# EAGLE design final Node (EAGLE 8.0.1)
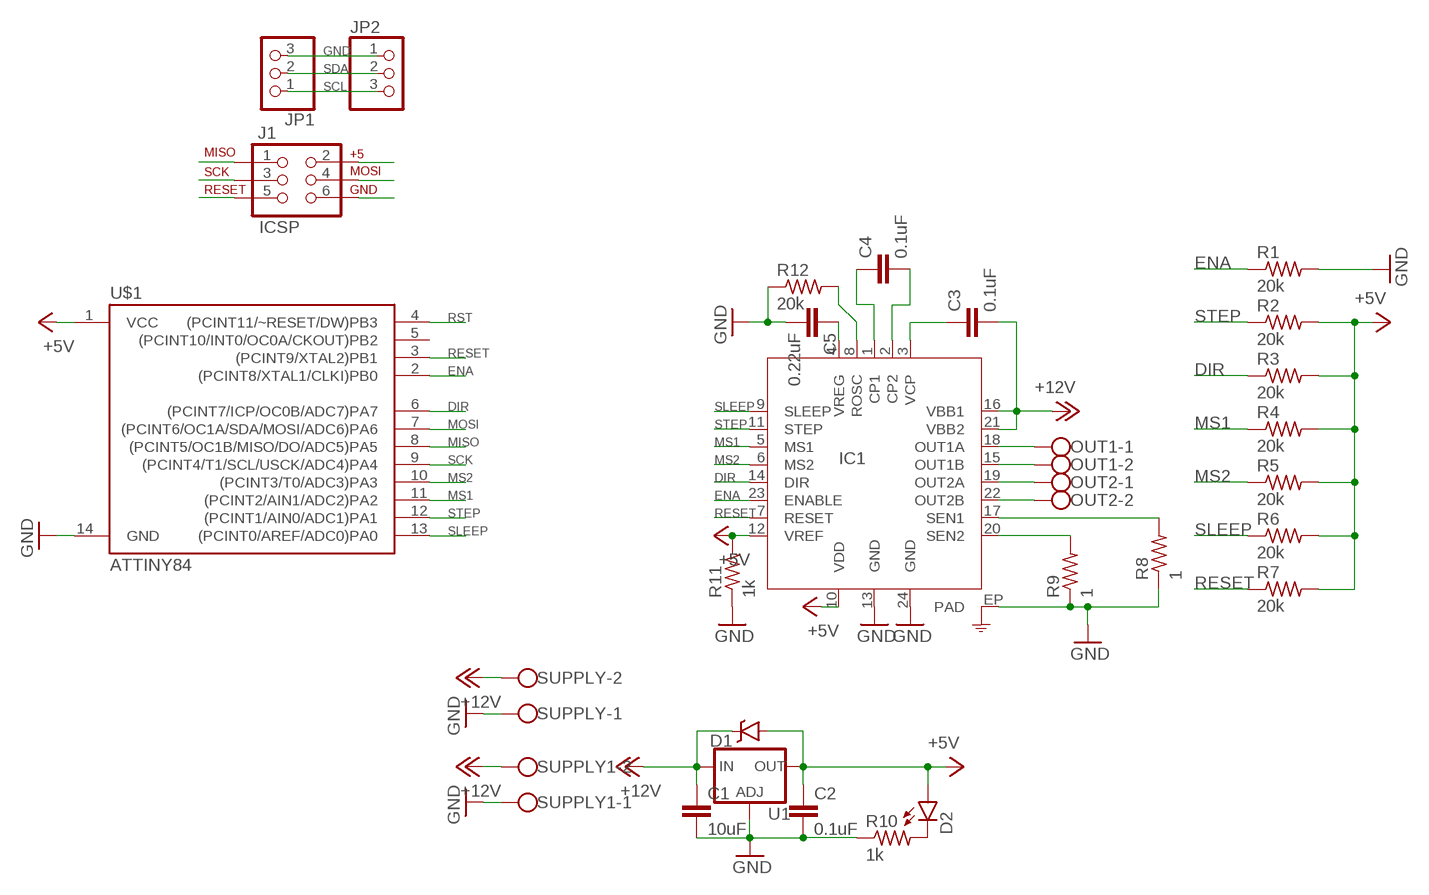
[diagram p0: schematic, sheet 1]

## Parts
C1  10uF  C-EUC1206  [C1206]
C2  0.1uF  C-EUC1206  [C1206]
C3  0.1uF  C-EUC1206  [C1206]
C4  0.1uF  C-EUC1206  [C1206]
C5  0.22uF  C-EUC1206  [C1206]
D1  DIODE-SCHOTTKY-BAT20J  [SOD-323]
D2  LED1206  [LED-1206]
IC1  A4982  [TSSOP-24]
J1  ICSP  AVR_SPI_PRG_6OFFSET_PADS  [2X3_OFFSET]
JP1  PINHD-1X3  [1X03]
JP2  PINHD-1X3  [1X03]
OUT1  W237-102  [W237-102]
OUT2  W237-102  [W237-102]
R1  20k  R-US_R1206  [R1206]
R2  20k  R-US_R1206  [R1206]
R3  20k  R-US_R1206  [R1206]
R4  20k  R-US_R1206  [R1206]
R5  20k  R-US_R1206  [R1206]
R6  20k  R-US_R1206  [R1206]
R7  20k  R-US_R1206  [R1206]
R8  1  R-US_R1206  [R1206]
R9  1  R-US_R1206  [R1206]
R10  1k  R-US_R1206  [R1206]
R11  1k  R-US_R1206  [R1206]
R12  20k  R-US_R1206  [R1206]
SUPPLY  W237-102  [W237-102]
SUPPLY1  W237-102  [W237-102]
U1  V_REG_317SMD  [SOT223]
U$1  ATTINY84  [SO14]

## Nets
5V: J1.2
+5V: C2.1 D1.A D2.A IC1.10(VDD) IC1.12(VREF) R2.2 R3.2 R4.2 R5.2 R6.2 R7.2 R11.2 U1.2(OUT) U$1.1(VCC)
+12V: C1.1 C3.2 D1.C IC1.16(VBB1) IC1.21(VBB2) SUPPLY1.2 SUPPLY.2 U1.3(IN)
DIR: IC1.14(DIR) R3.1 U$1.6((PCINT7/ICP/OC0B/ADC7)PA7)
ENA: IC1.23(ENABLE) R1.1 U$1.2((PCINT8/XTAL1/CLKI)PB0)
GND: C1.2 C2.2 C5.2 IC1.13(GND) IC1.24(GND) IC1.EP(PAD) J1.6 JP1.3 JP2.1 R1.2 R8.1 R9.1 R10.1 R11.1 R12.1 SUPPLY1.1 SUPPLY.1 U1.1(ADJ) U$1.14(GND)
MISO: J1.1 U$1.8((PCINT5/OC1B/MISO/DO/ADC5)PA5)
MOSI: J1.4 JP1.2 JP2.2 U$1.7((PCINT6/OC1A/SDA/MOSI/ADC6)PA6)
MS1: IC1.5(MS1) R4.1 U$1.11((PCINT2/AIN1/ADC2)PA2)
MS2: IC1.6(MS2) R5.1 U$1.10((PCINT3/T0/ADC3)PA3)
N$1: C3.1 IC1.3(VCP)
N$2: D2.C R10.2
N$8: C4.2 IC1.2(CP2)
N$9: C4.1 IC1.1(CP1)
N$11: C5.1 IC1.4(VREG)
N$12: IC1.8(ROSC) R12.2
OU1B: IC1.15(OUT1B) OUT1.2
OUT1A: IC1.18(OUT1A) OUT1.1
OUT2A: IC1.19(OUT2A) OUT2.1
OUT2B: IC1.22(OUT2B) OUT2.2
RESET: IC1.7(RESET) R7.1 U$1.3((PCINT9/XTAL2)PB1)
RST: J1.5 U$1.4((PCINT11/~RESET/DW)PB3)
SCK: J1.3 JP1.1 JP2.3 U$1.9((PCINT4/T1/SCL/USCK/ADC4)PA4)
SEN1: IC1.17(SEN1) R8.2
SEN2: IC1.20(SEN2) R9.2
SLEEP: IC1.9(SLEEP) R6.1 U$1.13((PCINT0/AREF/ADC0)PA0)
STEP: IC1.11(STEP) R2.1 U$1.12((PCINT1/AIN0/ADC1)PA1)
Unconnected: U$1.5((PCINT10/INT0/OC0A/CKOUT)PB2)

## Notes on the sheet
- SDA
- SCL

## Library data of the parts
C1-C5 = resistor:C-EU: CAPACITOR, European symbol
D1 = SparkFun-DiscreteSemi:DIODE-SCHOTTKY: Schottky diodes in SFE's production catalog; PROD_ID: DIO-11623; VALUE: BAT20J
D2 = SparkFun-LED:LED: LEDs
IC1 = SparkFun-DigitalIC:A4982: IC Full Bridge Motor Driver DMOS Microstepping Driver with Translator And Overcurrent Protection VBB 35V 2A
J1 = SparkFun-Connectors:AVR_SPI_PRG_6: AVR ISP 6 Pin This is the reduced ISP connector for AVR programming. Common on Arduino. This footprint will take up less PCB space and can be used with a 10-pin to 6-pin adapter such as SKU: BOB-08508 **Special note about "TEST_POINT" package. The stop mask is on the top side, so if you want your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
JP1 JP2 = pinhead:PINHD-1X3: PIN HEADER
OUT1 OUT2 SUPPLY SUPPLY1 = con-wago-500:W237-102: WAGO SCREW CLAMP; MPN: 237-102; OC_FARNELL: unknown; OC_NEWARK: 70K9898
R1-R12 = resistor:R-US_: RESISTOR, American symbol
U1 = SparkFun-PowerIC:V_REG_317: Voltage Regulator Standard LM317 adjustable voltage regulator. AOI (Adjust Output Input). Google 'LM317 Calculator' for easy to use app to get the two resistor values needed. 240/720 for 5V output. 240/390 for 3.3V output. Spark Fun Electronics SKU : COM-00527
U$1 = SparkFun-DigitalIC:ATTINY84: Atmel 14-pin 2/4/8kB flash uC; PROD_ID: IC-11285

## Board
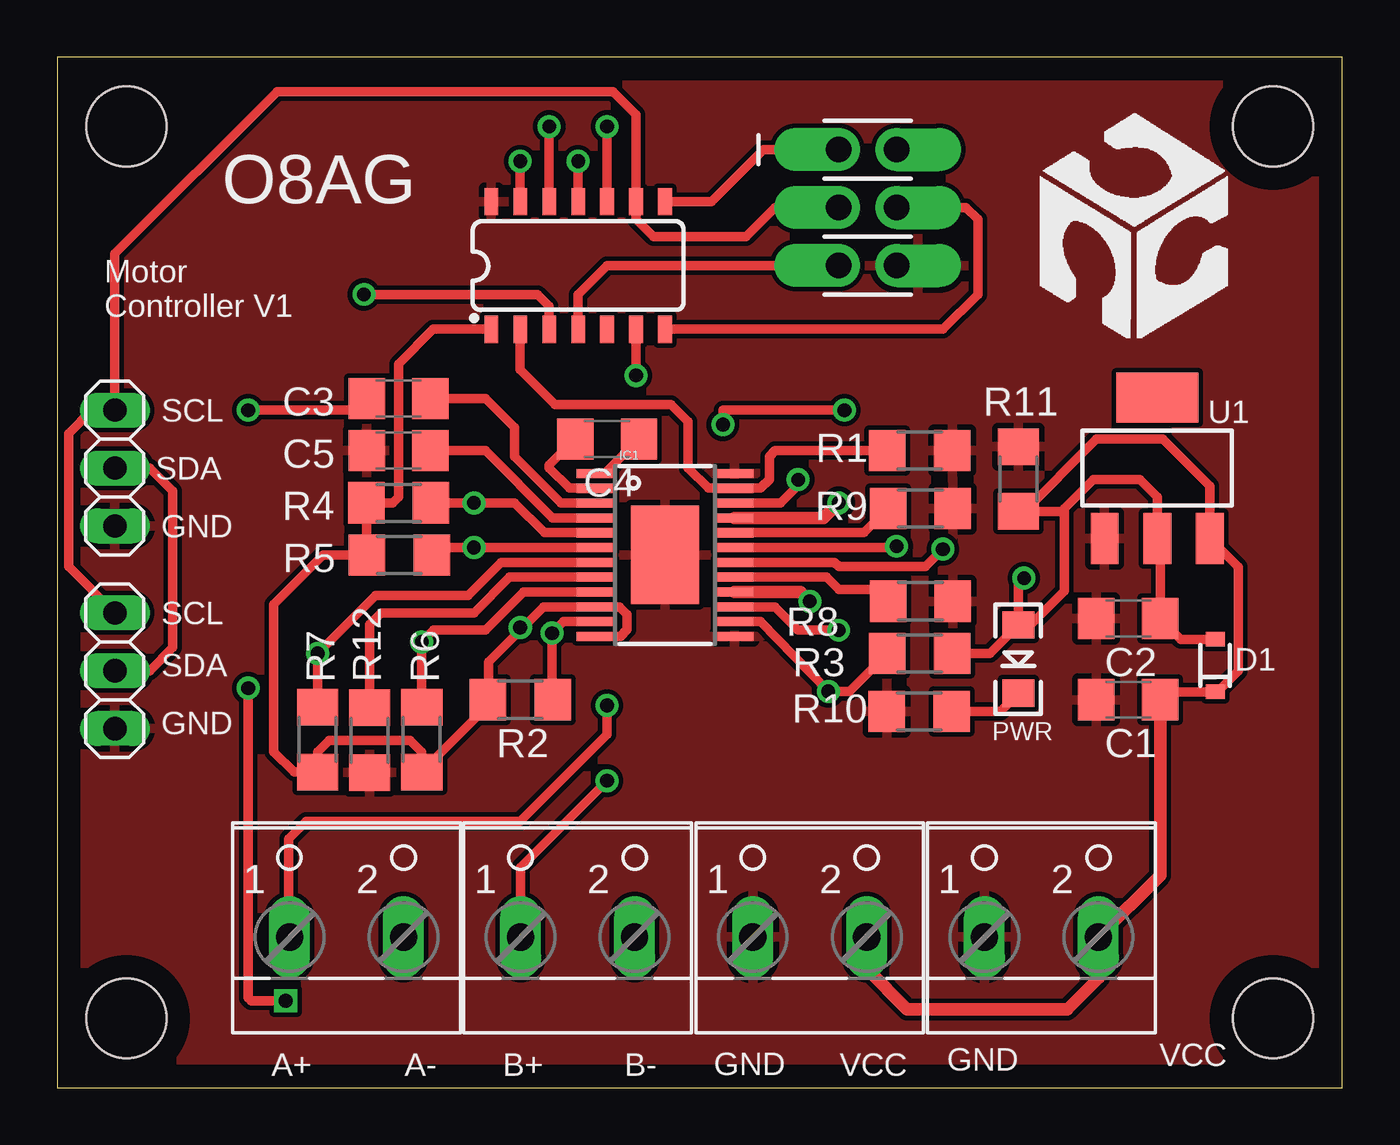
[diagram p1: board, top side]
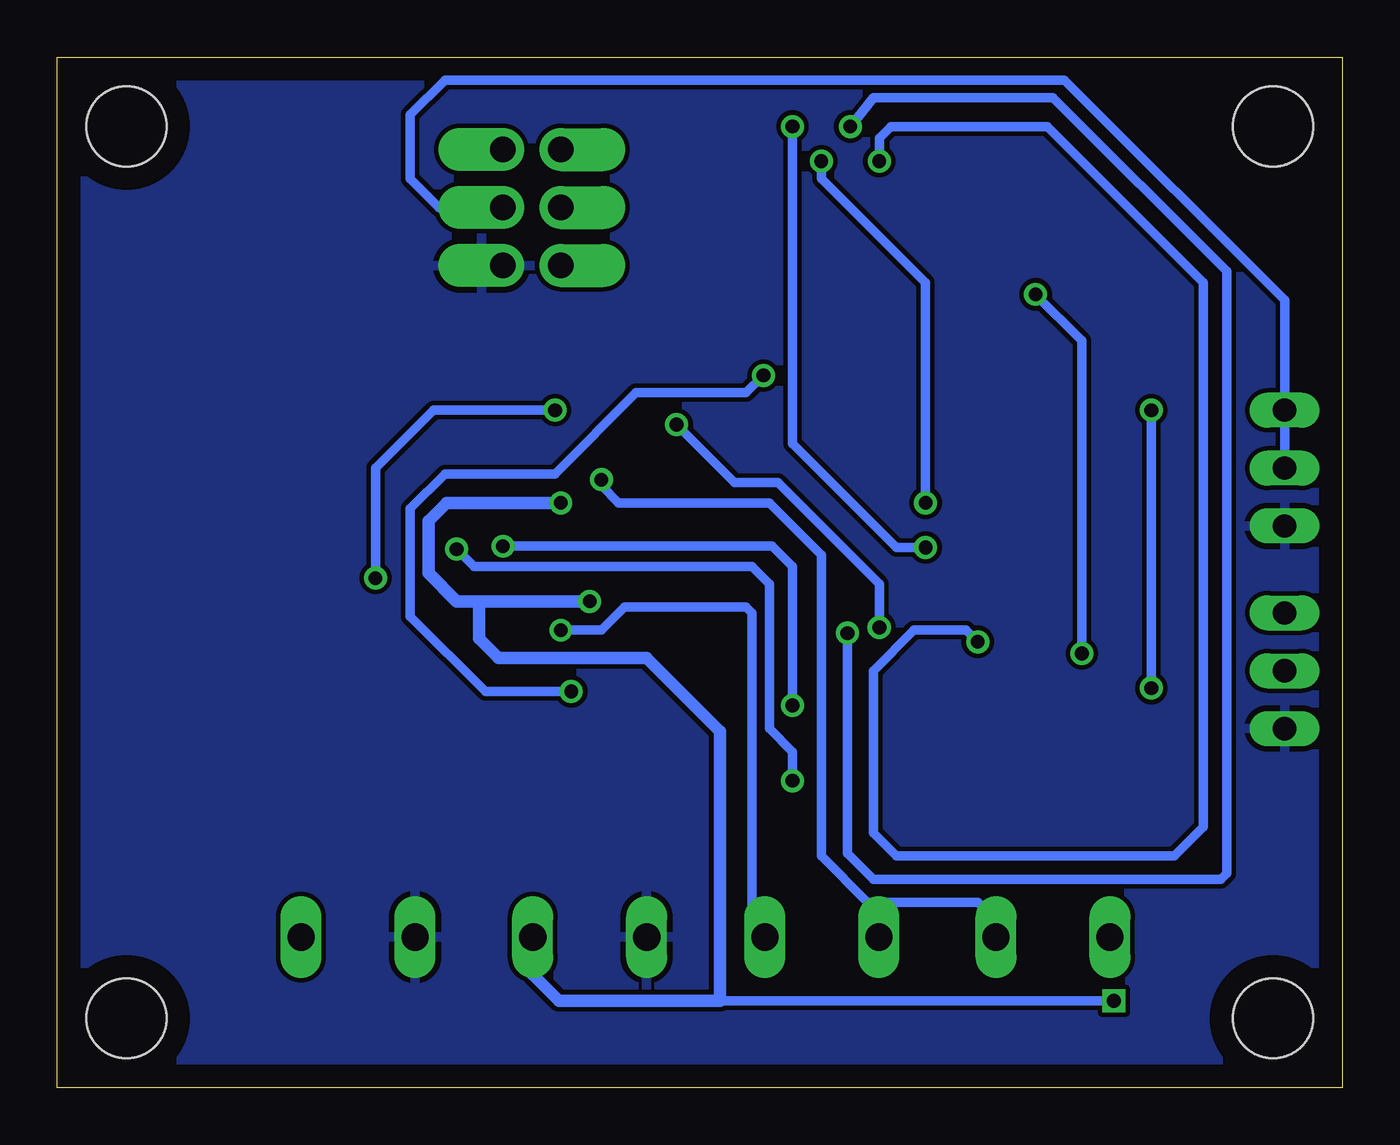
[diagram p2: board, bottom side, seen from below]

Size 56.39 x 45.21 mm. Coordinates in mm from the lower left corner, seen from the top.
Outline: 0,0 56.39,0 56.39,45.21 0,45.21 0,0
Copper layers (1*16): Top 0.035mm / dielectric 1.5mm / Bottom 0.035mm
Design rules "default *": minimum track width 16mil, minimum drill 24mil, track to track 8mil, track to pad 8mil, pad to pad 8mil, via to via 8mil, smd to smd 8mil, copper to edge 40mil, drill to drill 8mil, minimum pad ring 10mil, minimum via ring 8mil, stop-mask expansion 4mil, vias tented up to drill 0mil, thermal gap 10mil
Holes 3.5 mm at 3.05,3.05 53.34,3.05 53.34,42.16 3.05,42.16

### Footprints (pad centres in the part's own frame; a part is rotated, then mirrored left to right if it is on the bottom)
C1206 = smd 1.6 x 1.8: 1 -1.4,0; 2 1.4,0
SOD-323 = smd 0.63 x 0.83: A 1.15,0; C -1.15,0
LED-1206 = smd 1.2 x 1.4: A -1.5,0; C 1.5,0
TSSOP-24 = smd 0.4 x 1.65: 1 -3.575,-3.05; 2 -2.925,-3.05; 3 -2.275,-3.05; 4 -1.625,-3.05; 5 -0.975,-3.05; 6 -0.325,-3.05; 7 0.325,-3.05; 8 0.975,-3.05; 9 1.625,-3.05; 10 2.275,-3.05; 11 2.925,-3.05; 12 3.575,-3.05; 13 3.575,3.05; 14 2.925,3.05; 15 2.275,3.05; 16 1.625,3.05; 17 0.975,3.05; 18 0.325,3.05; 19 -0.325,3.05; 20 -0.975,3.05; 21 -1.625,3.05; 22 -2.275,3.05; 23 -2.925,3.05; 24 -3.575,3.05 | smd 4.32 x 3: EP 0,0
2X3_OFFSET = drill 1.118 pad 1.88 offset: 1 -2.54,-1.27; 2 -2.54,1.27; 3 0,-1.27; 4 0,1.27; 5 2.54,-1.27; 6 2.54,1.27
1X03 = drill 1.016 long: 1 -2.54,0; 2 0,0; 3 2.54,0
W237-102 = drill 1.194 long: 1 -2.5,-1.27; 2 2.5,-1.27
R1206 = smd 1.6 x 1.803: 1 -1.422,0; 2 1.422,0
SOT223 = smd 1.219 x 2.235: 1 -2.311,-3.099; 2 0,-3.099; 3 2.311,-3.099 | smd 3.6 x 2.2: 4 0,3.099
SO14 = smd 0.6 x 1.2: 1 -3.81,-2.8; 2 -2.54,-2.8; 3 -1.27,-2.8; 4 0,-2.8; 5 1.27,-2.8; 6 2.54,-2.8; 7 3.81,-2.8; 8 3.81,2.8; 9 2.54,2.8; 10 1.27,2.8; 11 0,2.8; 12 -1.27,2.8; 13 -2.54,2.8; 14 -3.81,2.8

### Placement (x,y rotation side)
C1  46.99,17.02 180 top
C2  46.99,20.57 180 top
C3  14.99,30.23 180 top
C4  24.13,28.45 180 top
C5  14.99,27.94 180 top
D1  50.8,18.52 90 top
D2  42.16,18.8 270 top
IC1  26.67,23.37 270 top
J1  35.56,38.61 270 top
JP1  2.54,27.18 270 top
JP2  2.54,18.29 90 top
OUT1  22.83,7.87 0 top
OUT2  12.7,7.87 0 top
R1  37.85,27.94 0 top
R2  20.32,17.02 180 top
R3  37.85,19.05 0 top
R4  14.99,25.65 180 top
R5  15.01,23.37 180 top
R6  16,15.27 270 top
R7  11.43,15.27 270 top
R8  37.87,21.34 180 top
R9  37.87,25.4 180 top
R10  37.82,16.51 0 top
R11  42.16,26.7 270 top
R12  13.72,15.24 90 top
SUPPLY  33.02,7.87 0 top
SUPPLY1  43.18,7.87 0 top
U1  48.26,27.18 0 top
U$1  22.86,36.07 0 top

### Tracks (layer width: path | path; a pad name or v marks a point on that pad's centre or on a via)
+5V  (via drill 0.6, 0.61)
  Top 0.406: 20.38,20.13 21.35,21.09 IC1.10 24.68,21.09 25.01,20.76 25.01,20.1 24.71,19.79 IC1.12 | 20.38,20.13 18.92,18.67 18.92,17.04 R2.2 18.9,16.74 R6.2 16,14.73 15.49,15.24 11.94,15.24 11.43,14.73 R7.2 | R7.2 10.4,13.84 9.51,14.73 9.51,21.19 11.68,23.37 R5.2 13.59,25.63 R4.2 14.73,25.65 14.99,25.91 14.99,31.75 16.5,33.27 U$1.1 | R7.2 | R3.2 40.92,19.05 D2.A | D2.A 42.7,20.3 44.2,21.8 44.2,24.88 | 48.51,20.45 C2.1 | D1.A 49.3,19.67 C2.1 | C2.1 48.39,23.95 U1.2 48.26,25.91 47.5,26.67 45.47,26.67 44.2,25.4 44.2,24.88 | v29.21,29.08 29.21,29.72 v34.54,29.72 | v20.32,20.19 20.38,20.13 | D2.A 42.16,22.1 v42.42,22.35 | 44.2,24.88 44.2,25.27 R11.2
  Bottom 0.406: v29.21,29.08 26.67,26.54 24.77,26.54 20.32,22.1 v20.32,20.19 | v42.42,22.35 42.42,27.18 39.88,29.72 v34.54,29.72
+12V  (via drill 0.6)
  Top 0.406: C1.1 48.74,17.37 D1.C 50.9,17.37 51.82,18.29 51.82,22.84 U1.3 50.57,26.39 48.51,28.45 45.59,28.45 42.29,25.15 | C3.2 13.34,29.72 v8.38,29.72 | 45.72,6.56 SUPPLY1.2 | v8.38,17.53 8.38,3.94 8.51,3.81 v10.03,3.81
  Top 0.559: SUPPLY.2 35.52,5.2 37.29,3.43 44.32,3.43 45.7,4.82 45.7,6.58 SUPPLY1.2 48.39,9.31 C1.1 | IC1.16 32.61,21.74 v33.02,21.34 | IC1.21 33.63,24.99 v34.29,25.65
  Top 0.711: SUPPLY1.2
  Bottom 0.406: 34.54,25.65 v34.29,25.65 | v10.03,3.81 27.3,3.81 | v8.38,29.72 v8.38,17.53
  Bottom 0.559: SUPPLY.2 35.51,6.59 35.51,4.95 34.37,3.81 27.3,3.81 27.3,15.62 30.53,18.84 37.03,18.84 37.88,19.7 37.88,21.34 38.05,21.34 | 38.05,21.34 38.86,21.34 40.09,22.57 40.09,24.85 39.29,25.65 v34.29,25.65 | 38.05,21.34 v33.02,21.34
DIR  (via drill 0.6)
  Top 0.406: 35.81,18.8 36.07,19.05 R3.1 34.75,17.38 v33.83,17.38 30.86,20.44 IC1.14 | v25.4,31.24 U$1.6
  Bottom 0.406: v33.83,17.38 37.59,17.38 40.89,20.68 40.89,25.4 39.37,26.92 34.54,26.92 30.99,30.48 26.16,30.48 v25.4,31.24
ENA
  Top 0.406: U$1.2 20.32,31.5 21.84,29.97 26.92,29.97 27.69,29.21 27.69,27.18 28.57,26.29 IC1.23 30.86,26.29 31.24,26.67 31.24,27.69 31.5,27.94 R1.1
GND
  pour Bottom: 0,-0.13 56.39,0.13 56.39,45.21 0,45.21
  pour Top: 0,-0.13 56.39,0.13 56.39,45.21 0,45.21
MISO
  Top 0.406: U$1.8 28.71,38.87 30.99,41.15 J1.1
MOSI
  Top 0.406: JP1.2 4.06,27.18 5.08,26.16 5.08,19.3 4.06,18.29 JP2.2 | J1.4 39.88,38.61 40.39,38.1 40.39,34.8 38.86,33.27 U$1.7
  Bottom 0.406: JP1.2 2.54,34.54 12.19,44.2 39.37,44.2 40.89,42.67 40.89,39.88 39.62,38.61 J1.4
MS1  (via drill 0.6)
  Top 0.406: IC1.5 21.38,24.34 20.07,25.65 v18.29,25.65 R4.1 | U$1.11 v22.86,40.64
  Bottom 0.406: v22.86,40.64 22.86,39.88 18.29,35.31 v18.29,25.65
MS2  (via drill 0.6)
  Top 0.406: IC1.6 v18.29,23.69 16.76,23.69 R5.1 | U$1.10 v24.13,42.16
  Bottom 0.406: v24.13,42.16 24.13,28.27 19.56,23.69 v18.29,23.69
N$1
  Top 0.406: IC1.3 22.11,25.64 20.07,27.69 20.07,28.96 18.8,30.23 C3.1
N$2
  Top 0.406: R10.2 41.38,16.51 D2.C
N$8
  Top 0.406: IC1.2 22.48,26.29 21.59,27.18 21.59,27.31 C4.2
N$9
  Top 0.406: IC1.1 24.02,26.94 C4.1
N$11
  Top 0.406: IC1.4 21.74,24.99 18.8,27.94 C5.1
N$12
  Top 0.406: IC1.8 19.85,22.39 18.29,20.83 14.22,20.83 13.72,20.32 R12.2
OU1B  (via drill 0.6)
  Top 0.406: IC1.15 31.48,21.09 32.51,20.07 v34.29,20.07
  Bottom 0.406: v34.29,20.07 32.51,20.07 31.5,21.08 26.16,21.08 25.91,20.83 25.91,7.43 OUT1.2
OUT1A  (via drill 0.6)
  Top 0.406: OUT1.1 20.34,9.67 v24.13,13.46 | v38.86,23.62 38.1,22.86 34.29,22.86 34.11,23.04 IC1.18
  Bottom 0.406: v24.13,13.46 24.13,14.73 25.15,15.75 25.15,22.1 25.91,22.86 38.1,22.86 v38.86,23.62
OUT2A  (via drill 0.6)
  Top 0.406: IC1.19 36.83,23.69 v36.83,23.75 | v24.13,16.76 24.13,15.49 20.32,11.68 10.92,11.68 10.16,10.92 10.16,6.39 OUT2.1
  Bottom 0.406: v36.83,23.75 25.02,23.75 24.13,22.86 v24.13,16.76
OUT2B  (via drill 0.6)
  Top 0.406: IC1.22 31.74,25.64 32.51,26.42 v32.51,26.67
  Bottom 0.406: v32.51,26.67 32.51,26.42 31.75,25.65 25.15,25.65 22.86,23.37 22.86,10.16 20.83,8.13 16,8.13 15.24,7.37 15.24,6.64 OUT2.2
RESET  (via drill 0.6)
  Top 0.406: R7.1 v11.43,19.05 13.97,21.59 18.03,21.59 19.49,23.04 IC1.7 | U$1.3 21.59,34.29 21.08,34.8 v13.46,34.8
  Bottom 0.406: v11.43,19.05 11.43,32.77 v13.46,34.8
RST
  Top 0.406: J1.5 24.13,36.07 22.86,34.8 U$1.4
SCK
  Top 0.406: J1.3 31.5,38.61 30.23,37.34 26.16,37.34 25.4,38.1 U$1.9 25.4,42.67 24.38,43.69 9.65,43.69 2.54,36.58 JP1.1 1.52,29.72 0.51,28.7 0.51,22.86 JP2.3
SEN1
  Top 0.406: IC1.17 33.74,22.39 34.29,21.84 35.94,21.84 R8.2
SEN2
  Top 0.406: IC1.20 35.39,24.34 R9.2
SLEEP  (via drill 0.6)
  Top 0.406: IC1.9 20.47,21.74 18.8,20.07 16.51,20.07 v16,19.56 R6.1 | U$1.13 v20.32,40.64
  Bottom 0.406: v20.32,40.64 20.32,41.66 19.81,42.16 12.95,42.16 6.1,35.31 6.1,11.43 7.37,10.16 19.56,10.16 20.57,11.18 20.57,18.29 18.8,20.07 16.51,20.07 v16,19.56
STEP  (via drill 0.6)
  Top 0.406: 21.84,17.02 R2.1 21.72,17.04 v21.72,19.94 22.22,20.44 IC1.11 | v21.59,42.16 U$1.12
  Bottom 0.406: v21.72,19.94 21.72,10.29 20.57,9.14 5.33,9.14 5.08,9.4 5.08,35.81 12.7,43.43 20.57,43.43 v21.59,42.16

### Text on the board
tNames: O8AG | Motor / Controller V1 | SCL | SDA | GND | SCL | SDA | GND | PWR | A+ | A- | B+ | B- | GND | VCC | GND | VCC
